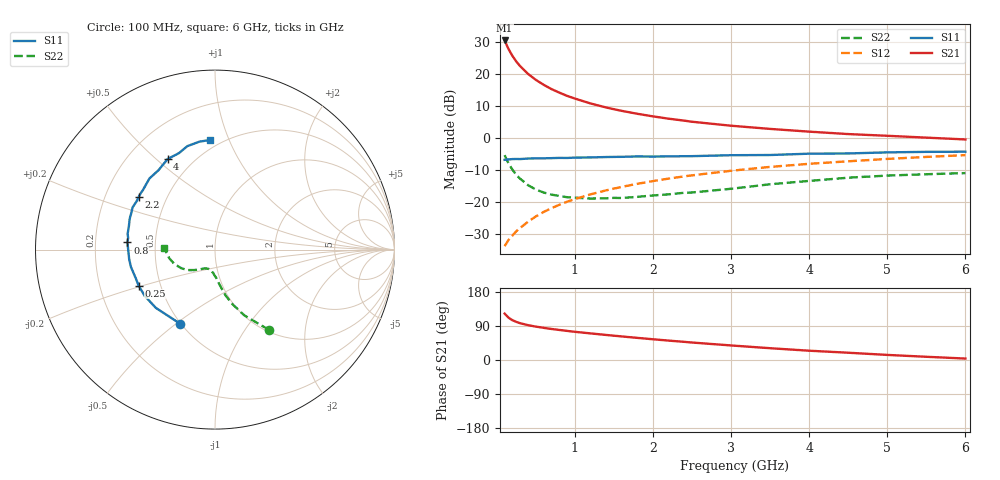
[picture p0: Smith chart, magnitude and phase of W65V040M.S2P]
! SIEMENS Small Signal Semiconductors
! BFR193W
! Si NPN RF Bipolar Junction Transistor in SOT323
! VCE = 5 V  IC = 40 mA
! Common Emitter S-Parameters:  September  1992
# GHz  S  MA  R  50
!  f  S11  S21  S12  S22
! GHz  MAG  ANG  MAG  ANG  MAG  ANG  MAG  ANG
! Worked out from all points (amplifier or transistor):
!   28 points, 100 MHz to 6 GHz, reference 50 ohm
!   highest |S21| = 30.5 dB at 100 MHz (marker M1)
!   |S21| within 3 dB of that: start of sweep to 157.5 MHz
!   unconditionally stable (mu >= 1): 592.6 MHz to 2.559 GHz
!   at 300 MHz: K = 0.89, MSG = 25.2 dB, |S12| = -28.0 dB
!   at 1.5 GHz: K = 1.03, MAG = 11.3 dB, |S12| = -15.8 dB
!   at 6 GHz: K = 0.92, MSG = 2.4 dB, |S12| = -5.3 dB
!   S11 on the Smith chart (normalised r, x): 100 MHz: 0.50, -0.52; 250 MHz: 0.38, -0.19; 800 MHz: 0.34, +0.04; 2.2 GHz: 0.35, +0.28; 4 GHz: 0.36, +0.54; 6 GHz: 0.44, +0.86
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0.1  0.4565 -115.0  33.31 122.5  0.0205 59.7  0.5402 -56.0
0.15  0.4627 -135.4  24.48 111.7  0.0256 60.6  0.4021 -65.9
0.2  0.4691 -146.8  19.14 105.0  0.03 61.9  0.3208 -72.1
0.25  0.4704 -154.7  15.62 100.5  0.0351 63.9  0.2654 -76.7
0.3  0.4694 -160.0  13.2 97.0  0.0396 65.9  0.2309 -79.4
0.4  0.4782 -168.3  10.02 92.0  0.0493 68.3  0.1836 -84.1
0.5  0.4812 -173.6  8.078 88.1  0.0597 70.1  0.1567 -87.7
0.6  0.4821 -177.9  6.769 84.9  0.0701 70.7  0.1411 -91.8
0.7  0.4851 178.6  5.803 81.9  0.0802 71.3  0.1307 -94.4
0.8  0.4894 175.3  5.109 79.3  0.0907 71.5  0.1249 -97.5
0.9  0.4882 172.4  4.548 76.8  0.1012 71.4  0.119 -99.7
1  0.4945 169.7  4.126 74.4  0.1114 71.1  0.1171 -102.0
1.2  0.4975 164.5  3.463 70.2  0.132 70.4  0.1135 -107.8
1.4  0.5047 160.5  2.996 66.1  0.1525 69.3  0.1144 -111.8
1.6  0.5084 156.7  2.653 62.2  0.1727 68.1  0.1158 -116.1
2.2  0.517 145.1  2.003 51.2  0.2324 63.9  0.132 -125.0
3  0.539 132.6  1.555 38.4  0.3081 57.3  0.1613 -135.0
3.5  0.5428 125.5  1.387 31.1  0.3542 52.9  0.1897 -143.0
4  0.5694 117.6  1.257 24.5  0.3958 48.5  0.2139 -150.8
4.5  0.574 110.4  1.152 19.2  0.4329 44.3  0.2402 -160.4
5.5  0.6079 98.1  1.014 8.5  0.5069 36.1  0.272 -176.8
6  0.611 92.5  0.949 3.8  0.5406 31.8  0.2832 178.7
